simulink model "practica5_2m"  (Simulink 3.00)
settings: Solver=ode45  StartTime=0.0  StopTime=10.0  RelTol=1e-3
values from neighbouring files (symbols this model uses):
  k1 = kp + kd/T    (= 4.6)    [practica5_2.m]    (also in practica5_3.m = 1/abs(evalfr(Gz,ri(1))))
  k2 = ki*T - 2*kd/T - kp    (= -8.5988)    [practica5_2.m]    (also in practica5_3.m = 1/abs(evalfr(Gz,ri(2))))
  k3 = kd/T    (= 4)    [practica5_2.m]
  T = 0.1    [practica5_2.m]    (also in practica5_3.m = 1; practica5_4.m = 0.5)

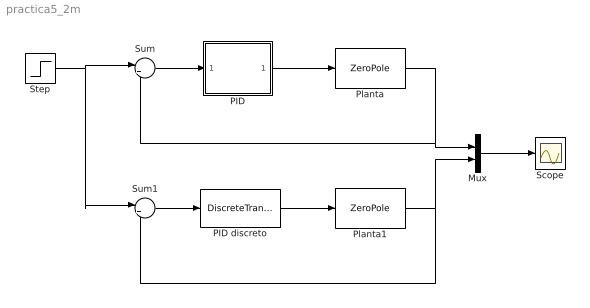
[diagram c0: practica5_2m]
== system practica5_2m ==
  Mux : Mux  Inputs=2
  PID : Subsystem
  PID discreto : DiscreteTransferFcn  Numerator=[k1 k2 k3]  Denominator=[1 -1 0]  SampleTime=T
  Planta : ZeroPole  Zeros=[]  Poles=[-1 -0.02]  Gain=[5]
  Planta1 : ZeroPole  Zeros=[]  Poles=[-1 -0.02]  Gain=[5]
  Scope : Scope
  Step : Step  Time=1  Before=0  After=1  SampleTime=0
  Sum : Sum  Inputs=|+-  SaturateOnIntegerOverflow=on
  Sum1 : Sum  Inputs=|+-  SaturateOnIntegerOverflow=on
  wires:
  PID/1(u) -> Planta/1
  Sum/1 -> PID/1(e)
  PID discreto/1 -> Planta1/1
  Sum1/1 -> PID discreto/1
  Step/1 -> Sum/1, Sum1/1
  Planta/1 -> Sum/2, Mux/1
  Planta1/1 -> Sum1/2, Mux/2
  Mux/1 -> Scope/1

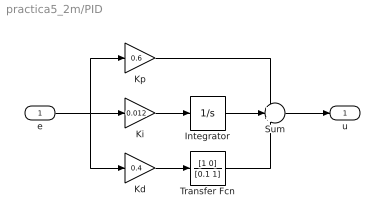
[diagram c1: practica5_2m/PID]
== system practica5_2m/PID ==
  e : Inport  Port=1  PortWidth=-1  SampleTime=-1  DataType=auto
  Integrator : Integrator  ExternalReset=none  InitialConditionSource=internal  InitialCondition=0  LimitOutput=off  UpperSaturationLimit=inf  LowerSaturationLimit=-inf  ShowSaturationPort=off  ShowStatePort=off  AbsoluteTolerance=auto
  Kd : Gain  Gain=0.4  SaturateOnIntegerOverflow=on
  Ki : Gain  Gain=0.012  SaturateOnIntegerOverflow=on
  Kp : Gain  Gain=0.6  SaturateOnIntegerOverflow=on
  Sum : Sum  Inputs=+++  SaturateOnIntegerOverflow=on
  Transfer Fcn : TransferFcn  Numerator=[1 0]  Denominator=[0.1 1]
  u : Outport  Port=1
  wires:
  Ki/1 -> Integrator/1
  Kd/1 -> Transfer Fcn/1
  Integrator/1 -> Sum/2
  Kp/1 -> Sum/1
  Transfer Fcn/1 -> Sum/3
  e/1 -> Ki/1, Kp/1, Kd/1
  Sum/1 -> u/1
